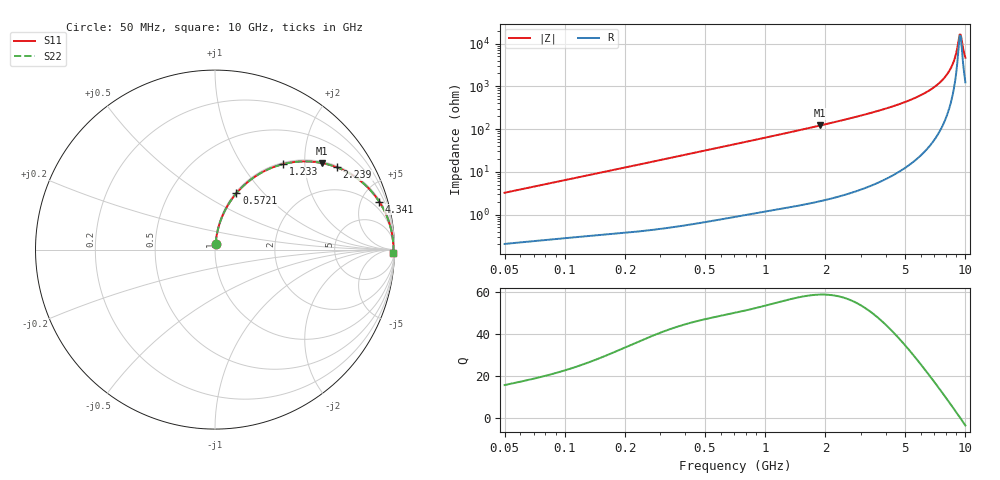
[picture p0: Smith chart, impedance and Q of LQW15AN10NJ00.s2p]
!Murata Part Number: LQW15AN10NJ00
!These Parameters are Measured in Series Mode Connection
!  o--[Z]--o
!Port1  Port2
!  o-------o
!Freq. Start=50[MHz] Stop=10[GHz], 401[Steps]
# Hz S RI R 50
!Freq.(Hz)	S 11(Real)	S 11(Imag)	S 21(Real)	S 21(Imag)	S 12(Real)	S 12(Imag)	S 22(Real)	S 22(Imag)
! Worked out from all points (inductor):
!   401 points, 50 MHz to 10 GHz, reference 50 ohm
!   read as one part in series: L = 10.2 nH near 51.34 MHz
!   highest Q = 59 at 1.884 GHz (marker M1), where L = 10.3 nH
!   self-resonance near 9.359 GHz
!   S11 on the Smith chart (normalised r, x): 50 MHz: 1.00, +0.06; 572.1 MHz: 1.01, +0.72; 1.233 GHz: 1.03, +1.56; 2.239 GHz: 1.05, +2.93; 4.341 GHz: 1.17, +6.80; 10 GHz: 26, -90
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5e7  0.00309 0.0322  0.9969 -0.0322  0.9969 -0.0322  0.00309 0.0322
1.214486e8  0.00891 0.0763  0.9911 -0.0763  0.9911 -0.0763  0.00891 0.0763
2.949953e8  0.0375 0.178  0.9625 -0.178  0.9625 -0.178  0.0375 0.178
5.720629e8  0.1192 0.3138  0.8808 -0.3138  0.8808 -0.3138  0.1192 0.3138
7.071068e8  0.1693 0.3652  0.8307 -0.3652  0.8307 -0.3652  0.1693 0.3652
1.233369e9  0.3794 0.4764  0.6206 -0.4764  0.6206 -0.4764  0.3794 0.4764
1.717543e9  0.5464 0.4894  0.4536 -0.4894  0.4536 -0.4894  0.5464 0.4894
1.884411e9  0.5942 0.4826  0.4058 -0.4826  0.4058 -0.4826  0.5942 0.4826
2.23851e9  0.6796 0.4581  0.3204 -0.4581  0.3204 -0.4581  0.6796 0.4581
4.171863e9  0.9057 0.2808  0.0943 -0.2808  0.0943 -0.2808  0.9057 0.2808
4.34098e9  0.9149 0.2671  0.0851 -0.2671  0.0851 -0.2671  0.9149 0.2671
6.045081e9  0.9699 0.152  0.0301 -0.152  0.0301 -0.152  0.9699 0.152
6.901252e9  0.9825 0.1062  0.0175 -0.1062  0.0175 -0.1062  0.9825 0.1062
7.571744e9  0.9885 0.0744  0.0115 -0.0744  0.0115 -0.0744  0.9885 0.0744
8.090191e9  0.9915 0.0518  0.00854 -0.0518  0.00854 -0.0518  0.9915 0.0518
8.530394e9  0.9931 0.0337  0.00693 -0.0337  0.00693 -0.0337  0.9931 0.0337
8.876195e9  0.9938 0.0202  0.00616 -0.0202  0.00616 -0.0202  0.9938 0.0202
9.236013e9  0.9942 0.00664  0.00576 -0.00664  0.00576 -0.00664  0.9942 0.00664
9.359165e9  0.9943 0.00213  0.00571 -0.00213  0.00571 -0.00213  0.9943 0.00213
9.48396e9  0.9943 -0.00237  0.0057 0.00237  0.0057 0.00237  0.9943 -0.00237
9.610418e9  0.9943 -0.00688  0.00574 0.00688  0.00574 0.00688  0.9943 -0.00688
1e10  0.9939 -0.0204  0.00608 0.0204  0.00608 0.0204  0.9939 -0.0204
